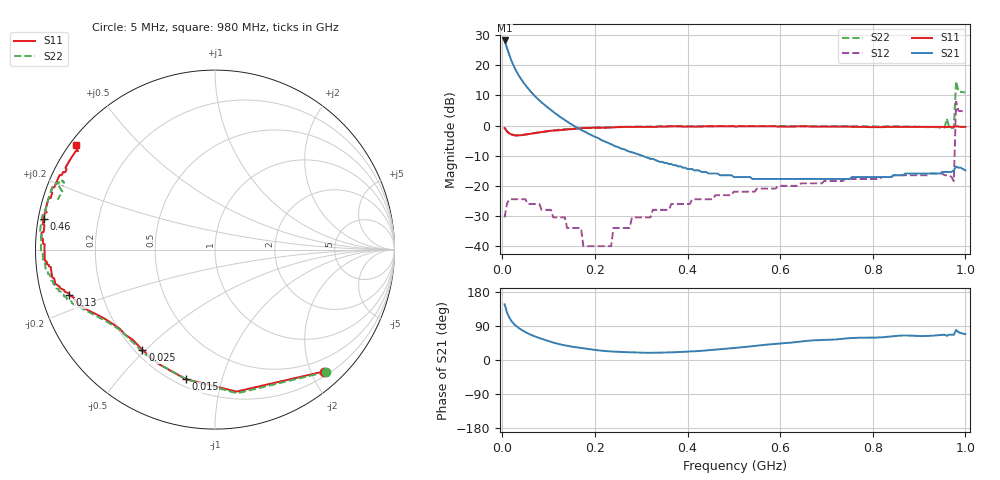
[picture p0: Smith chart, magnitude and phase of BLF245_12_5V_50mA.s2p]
! Filename:  BLF245_12.5V_50mA.s2p
! Philips part #: BLF245  !date: 22-05-2003
!Vdd=12.5V ; Idq=50 mA
!D:\Vee measurements\measurement data\VDMOST\BLF245\12.5V_50mA_#1
# HZ S MA R 50
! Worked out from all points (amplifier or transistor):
!   200 points, 5 MHz to 1 GHz, reference 50 ohm
!   highest |S21| = 28.2 dB at 5 MHz (marker M1)
!   |S21| within 3 dB of that: start of sweep to 11.22 MHz
!   unconditionally stable (mu >= 1): 175 MHz to 192.5 MHz; 206.3 MHz to 236.6 MHz; 610.6 MHz to 955.6 MHz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
!   at 170 MHz: K = 0.27, MSG = 16.3 dB, |S12| = -34.0 dB
!   at 505 MHz: K = 0.83, MSG = 2.4 dB, |S12| = -21.9 dB
!   at 1 GHz: K = -2.24, MSG = -9.8 dB, |S12| = 4.6 dB
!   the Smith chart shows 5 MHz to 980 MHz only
!   S11 on the Smith chart (normalised r, x): 5 MHz: 0.28, -2.20; 15 MHz: 0.24, -0.77; 25 MHz: 0.23, -0.49; 130 MHz: 0.08, -0.15; 460 MHz: 0.02, +0.09; 980 MHz: 0.02, +0.33
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5000000  0.91 -48.3  25.72 147.1  0.03 57.9  0.92 -47.8
1e7  0.8 -81.4  19.43 125.8  0.05 36.8  0.81 -81.3
1.5e7  0.74 -102.8  14.9 112.0  0.06 23.5  0.74 -102.4
2e7  0.71 -116.7  11.79 102.4  0.06 15.0  0.71 -115.5
2.5e7  0.69 -125.9  9.6 95.3  0.06 8.5  0.7 -124.7
4e7  0.69 -140.3  5.97 80.8  0.06 -4.4  0.69 -139.0
6e7  0.73 -148.6  3.76 67.5  0.05 -14.8  0.73 -147.2
9e7  0.79 -155.1  2.24 53.7  0.04 -23.8  0.79 -154.2
1.3e8  0.85 -162.6  1.31 39.9  0.03 -27.6  0.86 -160.8
1.75e8  0.91 -167.9  0.81 30.8  0.01 -8.4  0.91 -166.3
3.4e8  0.96 177.6  0.25 19.4  0.04 85.7  0.97 -179.3
4.6e8  0.97 170.0  0.16 27.2  0.07 86.2  0.97 174.5
5.05e8  0.96 167.5  0.14 32.2  0.08 84.5  0.98 172.4
6.7e8  0.96 158.6  0.13 51.8  0.11 81.4  0.97 165.6
8.35e8  0.95 151.0  0.14 61.6  0.14 80.2  0.97 159.2
9.5e8  0.95 144.9  0.17 66.3  0.16 74.1  0.93 155.7
9.6e8  0.94 144.3  0.17 63.6  0.15 -142.2  1.3 -171.2
9.65e8  0.95 144.2  0.17 66.8  0.15 74.9  0.94 157.8
9.75e8  0.95 143.7  0.18 66.5  0.12 69.6  0.92 162.4
9.8e8  0.97 143.2  0.21 79.3  2.49 39.9  5.44 42.2
9.85e8  0.96 143.1  0.2 73.5  1.76 41.6  3.67 47.3
1e9  0.95 142.7  0.18 68.2  1.7 40.5  3.52 46.0
